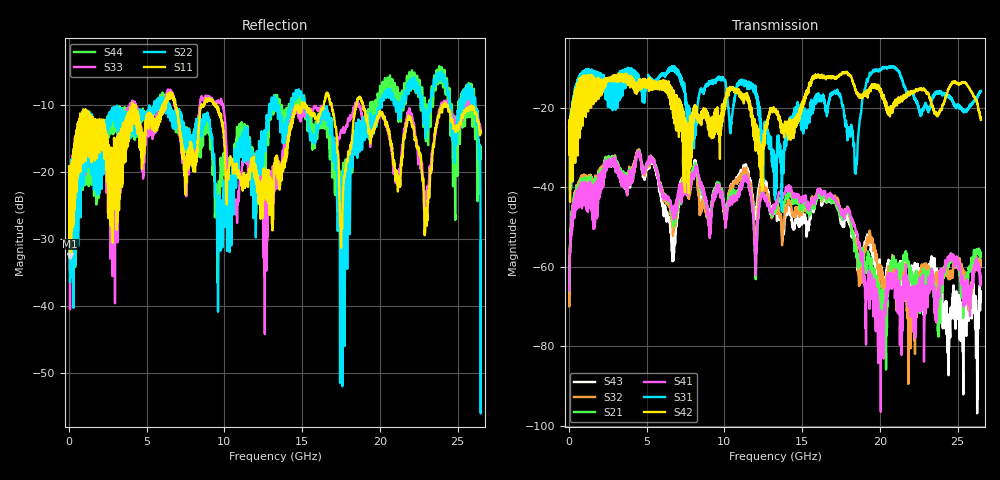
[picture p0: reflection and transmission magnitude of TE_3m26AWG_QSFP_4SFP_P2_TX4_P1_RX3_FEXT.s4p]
!Agilent Technologies,N5222A,MY51421691,A.10.00.00
!Agilent N5222A: A.10.00.00
!Date: Friday, January 30, 2015 12:37:03
!Correction: S11(Full 4 Port(1,2,3,4))
!S12(Full 4 Port(1,2,3,4))
!S13(Full 4 Port(1,2,3,4))
!S14(Full 4 Port(1,2,3,4))
!S21(Full 4 Port(1,2,3,4))
!S22(Full 4 Port(1,2,3,4))
!S23(Full 4 Port(1,2,3,4))
!S24(Full 4 Port(1,2,3,4))
!S31(Full 4 Port(1,2,3,4))
!S32(Full 4 Port(1,2,3,4))
!S33(Full 4 Port(1,2,3,4))
!S34(Full 4 Port(1,2,3,4))
!S41(Full 4 Port(1,2,3,4))
!S42(Full 4 Port(1,2,3,4))
!S43(Full 4 Port(1,2,3,4))
!S44(Full 4 Port(1,2,3,4))
!S4P File: Measurements: <S11,S12,S13,S14>,
!<S21,S22,S23,S24>,
!<S31,S32,S33,S34>,
!<S41,S42,S43,S44>:
# Hz S  dB  R 50.0
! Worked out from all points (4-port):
!   2650 points, 10 MHz to 26.5 GHz, reference 50 ohm
!   strongest paths, dB at 10 MHz, 6.63 GHz, 13.26 GHz, 19.88 GHz, 26.5 GHz:
!     S42: -25.0, -15.9, -20.3, -14.2, -23.0
!     S31: -24.9, -10.5, -43.1, -10.4, -15.7
!     S41: -65.4, -44.9, -45.1, -80.1, -62.4
!     S21: -66.0, -45.8, -46.5, -65.8, -56.4
!     S32: -60.4, -47.8, -45.2, -61.0, -58.2
!     S43: -63.2, -52.7, -45.3, -60.1, -66.2
!   lowest |S11| = -32.5 dB at 70 MHz (marker M1), VSWR 1.05, Z = 52.4 + j0.259 ohm
!   |S11| at or under -10 dB: start of sweep to 4.075 GHz; 9.454 GHz to 14.73 GHz (5.274 GHz wide, 43.6 % of centre); 18.91 GHz to 24.02 GHz (5.106 GHz wide, 23.8 % of centre)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
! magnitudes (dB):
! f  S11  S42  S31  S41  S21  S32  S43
! 10 MHz  -19.2  -25.0  -24.9  -65.4  -66.0  -60.4  -63.2
! 70 MHz  -32.5  -43.6  -40.7  -56.1  -55.1  -54.3  -54.9
! 4.46 GHz  -11.5  -13.8  -11.7  -31.9  -31.8  -31.5  -32.0
! 6.7 GHz  -8.8  -19.3  -10.5  -45.3  -46.7  -49.9  -52.9
! 13.22 GHz  -18.7  -20.5  -42.0  -44.8  -45.5  -45.6  -45.8
! 20.33 GHz  -12.3  -18.2  -9.8  -69.5  -67.2  -63.2  -64.1
! 26.5 GHz  -14.0  -23.0  -15.7  -62.4  -56.4  -58.2  -66.2
